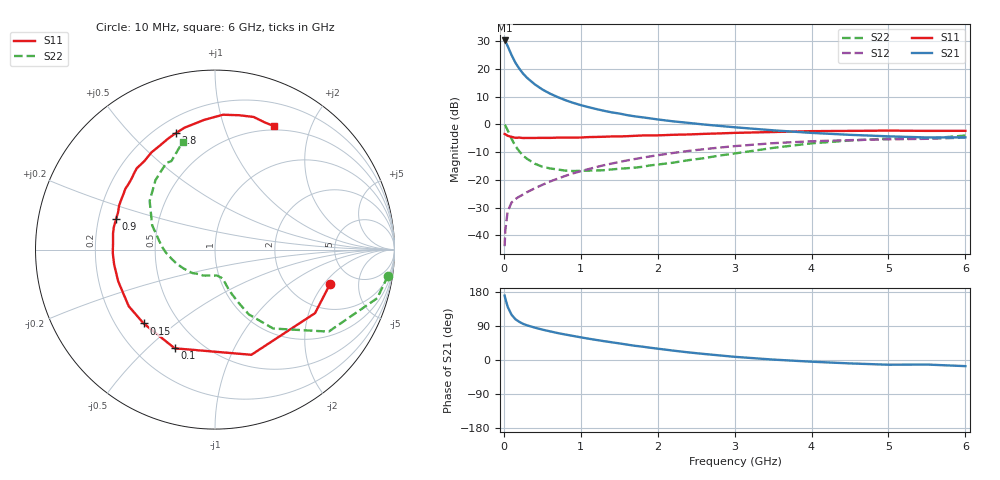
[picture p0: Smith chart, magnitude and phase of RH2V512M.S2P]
! SIEMENS Small Signal Semiconductors
! BFR106
! Si NPN RF Bipolar Junction Transistor in SOT23
! VCE = 2.5 V  IC = 12 mA
! Common Emitter S-Parameters:  August  1996
# GHz  S  MA  R  50
!  f  S11  S21  S12  S22
! GHz  MAG  ANG  MAG  ANG  MAG  ANG  MAG  ANG
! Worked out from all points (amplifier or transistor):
!   36 points, 10 MHz to 6 GHz, reference 50 ohm
!   highest |S21| = 30.2 dB at 10 MHz (marker M1)
!   |S21| within 3 dB of that: start of sweep to 64.96 MHz
!   unconditionally stable (mu >= 1): 446.5 MHz to 2.272 GHz; 5.007 GHz to end of sweep
!   at 250 MHz: K = 0.78, MSG = 21.8 dB, |S12| = -25.3 dB
!   at 1.4 GHz: K = 1.09, MAG = 7.4 dB, |S12| = -14.1 dB
!   at 6 GHz: K = 1.02, MAG = -0.7 dB, |S12| = -4.8 dB
!   S11 on the Smith chart (normalised r, x): 10 MHz: 3.34, -2.31; 100 MHz: 0.36, -0.61; 150 MHz: 0.32, -0.39; 900 MHz: 0.27, +0.14; 2.8 GHz: 0.28, +0.68; 6 GHz: 0.45, +1.49
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0.01  0.6691 -16.6  32.27 170.0  0.0064 84.4  0.975 -8.6
0.02  0.6604 -32.4  31.2 161.7  0.0127 75.6  0.9432 -16.7
0.05  0.6201 -70.9  25.49 140.1  0.027 60.7  0.7811 -35.8
0.1  0.5941 -112.2  17.68 119.5  0.0391 50.0  0.5465 -53.6
0.15  0.5722 -134.0  12.87 107.6  0.0451 46.1  0.4074 -62.4
0.2  0.5749 -146.7  10.08 100.8  0.0499 47.0  0.3276 -65.9
0.25  0.566 -155.7  8.171 95.4  0.0545 48.4  0.272 -68.8
0.3  0.5674 -162.2  6.896 91.6  0.0599 50.5  0.2404 -70.8
0.4  0.568 -171.6  5.263 85.6  0.0702 54.1  0.1961 -73.0
0.5  0.5698 -178.1  4.234 80.2  0.0812 56.8  0.1723 -74.6
0.6  0.5693 176.3  3.564 75.6  0.0932 58.6  0.1607 -77.3
0.7  0.5752 170.9  3.088 71.1  0.1051 59.9  0.1533 -80.9
0.9  0.577 162.9  2.435 63.5  0.1307 60.8  0.144 -87.2
1.1  0.588 155.3  2.035 56.3  0.1561 60.5  0.1467 -96.1
1.3  0.5966 148.7  1.751 49.8  0.1832 59.5  0.149 -105.0
1.6  0.6102 139.6  1.464 40.7  0.2232 57.0  0.1618 -119.8
2.2  0.647 123.2  1.13 24.8  0.3045 49.8  0.2036 -148.7
2.8  0.685 108.5  0.936 12.2  0.3803 40.8  0.2732 -176.3
3.5  0.7257 94.6  0.779 1.1  0.4568 29.5  0.3757 158.8
4.5  0.7605 79.9  0.646 -9.0  0.5184 13.3  0.5101 130.5
5.5  0.7608 68.5  0.579 -12.0  0.5478 3.1  0.5499 116.2
6  0.7627 64.5  0.582 -16.2  0.575 -4.3  0.6276 106.6
